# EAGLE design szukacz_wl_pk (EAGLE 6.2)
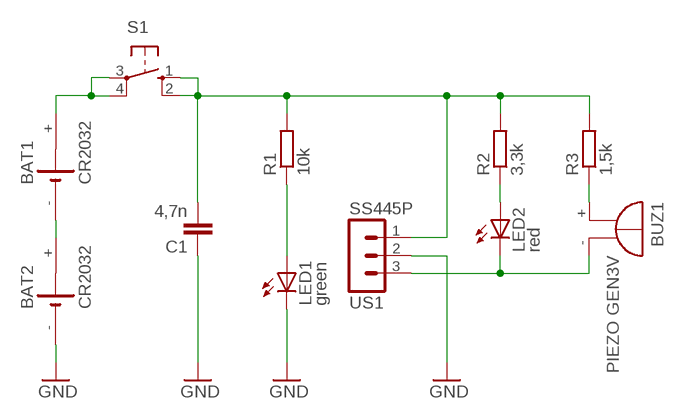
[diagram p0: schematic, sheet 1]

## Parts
BAT1  CR2032  BAT_20/16_XX  [BAT_CR2032]
BAT2  CR2032  BAT_20/16_XX  [BAT_CR2032]
BUZ1  PIEZO GEN3V  F/TMB  [F/TMB]
C1  4,7n  C-EU050-025X075  [C050-025X075]
LED1  green  LED5MM  [LED5MM]
LED2  red  LED5MM  [LED5MM]
R1  10k  R-EU_0207/7  [0207/7]
R2  3,3k  R-EU_0207/7  [0207/7]
R3  1,5k  R-EU_0207/7  [0207/7]
S1  40-XX  [B3F-40XX]
US1  SS445P  MA03-1  [MA03-1]

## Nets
GND: BAT2.- C1.1 LED1.K(C) US1.2
N$1: BAT1.+ S1.3(P) S1.4(P1)
N$2: BAT1.- BAT2.+
N$3: C1.2 R1.2 R2.2 R3.2 S1.1(S) S1.2(S1) US1.1
N$4: LED1.A R1.1
N$5: BUZ1.- LED2.K(C) US1.3
N$6: LED2.A R2.1
N$7: BUZ1.+ R3.1

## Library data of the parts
BAT1 BAT2 = inne_futrzak:BAT_20/16_XX
BUZ1 = buzzer:F/TMB: BUZZER; OC_FARNELL: unknown; OC_NEWARK: unknown
C1 = rcl:C-EU: CAPACITOR, European symbol
LED1 LED2 = led:LED: LED
R1-R3 = rcl:R-EU_: RESISTOR, European symbol
S1 = switch-omron:40-XX: OMRON SWITCH; MF: OMRON COMPONENTS USA; MPN: B3F-4000; OC_FARNELL: 176434; OC_NEWARK: 36K3105
US1 = con-lstb:MA03-1: PIN HEADER; OC_FARNELL: unknown; OC_NEWARK: unknown

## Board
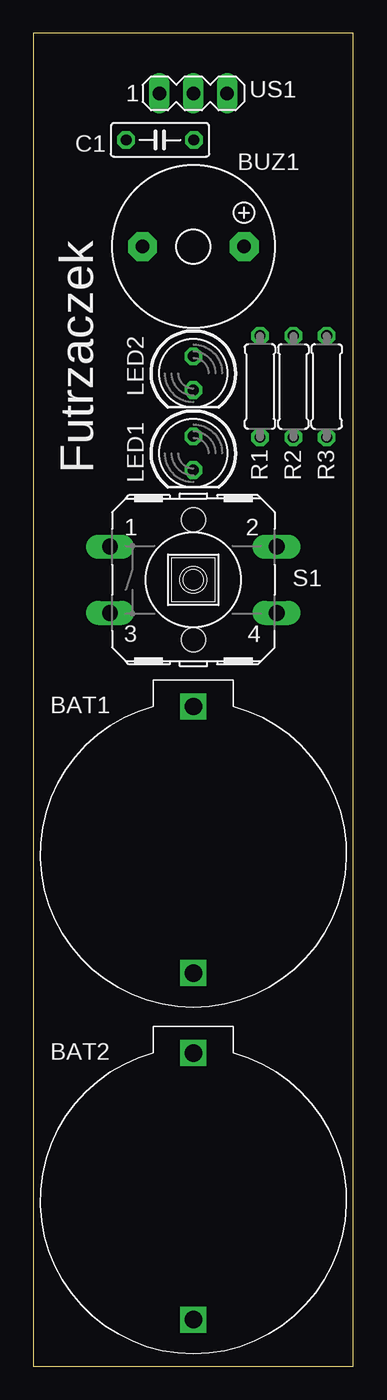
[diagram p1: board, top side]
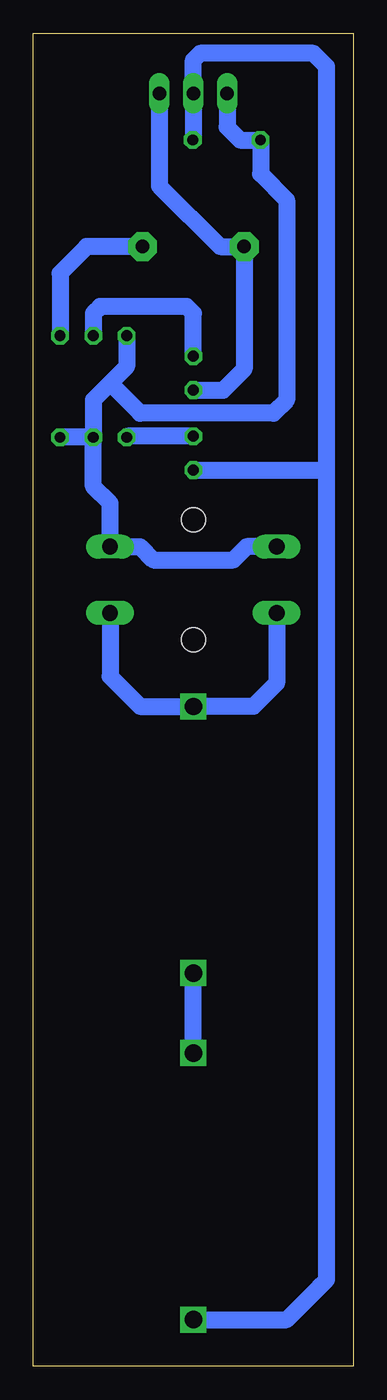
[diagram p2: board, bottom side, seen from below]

Size 24 x 100 mm. Coordinates in mm from the lower left corner, seen from the top.
Outline: 0,0 24,0 24,100 0,100 0,0
Copper layers (1*16): Top 0.035mm / dielectric 1.5mm / Bottom 0.035mm
Design rules: minimum track width 10mil, minimum drill 24mil, track to track 8mil, track to pad 8mil, pad to pad 8mil, via to via 8mil, smd to smd 8mil, copper to edge 20mil, drill to drill 8mil, minimum pad ring 10mil, minimum via ring 8mil, stop-mask expansion 4mil, vias tented up to drill 0mil, thermal gap 10mil

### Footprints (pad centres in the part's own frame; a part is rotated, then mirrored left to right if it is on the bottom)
BAT_CR2032 = drill 1.3 square: + 12,0; - -8,0
F/TMB = drill 1.016 pad 2.159 octagon: + 3.81,0; - -3.81,0
C050-025X075 = drill 0.813 octagon: 1 -2.54,0; 2 2.54,0
LED5MM = drill 0.813 octagon: A -1.27,0; K 1.27,0
0207/7 = drill 0.813 octagon: 1 -3.81,0; 2 3.81,0
B3F-40XX = drill 1.194 long: 1 -6.248,2.489; 2 6.248,2.489; 3 -6.248,-2.489; 4 6.248,-2.489 | hole 1.803: 0,-4.496; 0,4.496
MA03-1 = drill 1.016 long: 1 -2.54,0; 2 0,0; 3 2.54,0

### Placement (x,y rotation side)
BAT1  12,37.5 90 top
BAT2  12,11.5 90 top
BUZ1  12,84 0 top
C1  9.5,92 180 top
LED1  12,68.5 270 top
LED2  12,74.5 270 top
R1  17,73.5 90 top
R2  19.5,73.5 270 top
R3  22,73.5 270 top
S1  12,59 0 top
US1  12,95.5 0 top

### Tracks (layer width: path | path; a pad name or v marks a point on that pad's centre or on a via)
GND
  Bottom 1.27: BAT2.- 5,3.5 2.5,6 2,6.5 2,67 | 2,67 2,89 2,97.5 3,98.5 11.5,98.5 12,98 US1.2 12,92.04 C1.1 | LED1.K 2.23,67.23 2,67
N$1
  Bottom 1.27: S1.3 5.75,51.25 7.5,49.5 BAT1.+ 16,49.5 18.25,51.75 S1.4
N$2
  Bottom 1.27: BAT2.+ BAT1.-
N$3
  Bottom 1.27: R2.2 19.5,66 18.25,64.75 S1.2 15.99,61.49 15,60.5 9,60.5 8.01,61.49 S1.1 | R2.2 R3.2 | R1.2 17,75 18.25,73.75 | 18.25,73.75 19.5,72.5 R2.2 | US1.1 9.46,92.96 8.5,92 C1.2 6.96,89.46 5,87.5 5,72.5 6,71.5 16,71.5 18.25,73.75
N$4
  Bottom 1.27: LED1.A 16.92,69.77 R1.1
N$5
  Bottom 1.27: US1.3 14.54,88.54 10,84 BUZ1.- 8.19,74.81 8.5,74.5 9.77,73.23 LED2.K
N$6
  Bottom 1.27: LED2.A 12,79 12.5,79.5 19,79.5 19.5,79 R2.1
N$7
  Bottom 1.27: BUZ1.+ 20,84 22,82 R3.1

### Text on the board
tPlace: Futrzaczek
